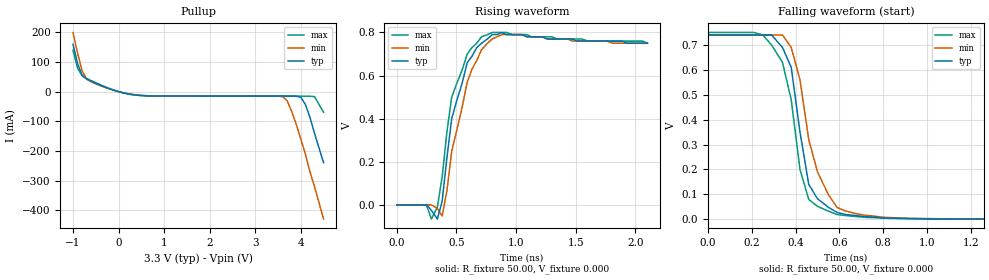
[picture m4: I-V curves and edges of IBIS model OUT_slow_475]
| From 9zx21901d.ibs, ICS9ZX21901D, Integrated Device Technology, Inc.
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|   Model OUT_slow_475
[Model]   OUT_slow_475
Model_type   Open_source
Polarity   Non-Inverting
Enable   Active-High
Vmeas =  0.350V
Cref =   2.00pF
Rref =  83.000
Vref =   0.350V
C_comp   3.40pF   2.85pF   3.95pF
[Temperature Range]   27.00   70.00   0.000
[Voltage Range]   3.30V   3.00V   3.60V
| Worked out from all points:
|   slope of the pullup table from 0 to 0.495 V, typ, clamps not added: 38 ohm
|   rising waveform, R_fixture 50.00, V_fixture 0.000: 20-80 % time 157ps typ, 172ps min, 145ps max; typ from 0.001 V to 0.75 V
|   falling waveform, R_fixture 50.00, V_fixture 0.000: 20-80 % time 75.6ps typ, 113ps min, 88.4ps max; typ from 0.74 V to 0.001 V
[Pullup]
| voltage   I(typ)   I(min)   I(max)
| -3.30   2.07A   2.09A   2.05A
| -3.10   1.90A   1.92A   1.88A
| -2.90   1.73A   1.75A   1.71A
| -2.70   1.56A   1.58A   1.54A
| -2.50   1.39A   1.42A   1.37A
| -2.30   1.22A   1.25A   1.20A
| -2.10   1.05A   1.08A   1.03A
| -1.90   0.89A   0.92A   0.87A
| -1.70   0.72A   0.75A   0.70A
| -1.50   0.56A   0.59A   0.53A
-1V       160mA      200mA      140mA
-900mV    95.74mA    130mA      79.64mA
-800mV    55.08mA    70.81mA    53.91mA
-700mV    42.76mA    42.1mA     45.09mA
-100mV    4.89mA     4.52mA     5.18mA
600mV     -13.67mA   -13.38mA   -13.83mA
3.6V      -14.91mA   -16.65mA   -14.97mA
3.8V      -14.95mA   -66.77mA   -14.97mA
4V        -18.98mA   -160mA     -14.97mA
4.1V      -42.81mA   -210mA     -14.99mA
4.3V      -140mA     -320mA     -16.63mA
4.5V      -240mA     -430mA     -69.57mA
|  4.70   -0.35A   -0.54A   -0.17A
|  4.90   -0.47A   -0.65A   -0.28A
|  5.10   -0.58A   -0.76A   -0.40A
|  5.30   -0.70A   -0.88A   -0.51A
|  5.50   -0.81A   -0.99A   -0.63A
|  5.70   -0.92A   -1.10A   -0.75A
|  5.90   -1.04A   -1.21A   -0.86A
|  6.10   -1.15A   -1.33A   -0.98A
|  6.60   -1.44A   -1.61A   -1.27A
[Ramp]
| variable   typ   min   max
dV/dt_r   0.45/0.16n   0.45/0.17n   0.45/0.16n
dV/dt_f   0.45/96.18p   0.45/0.11n   0.45/89.65p
R_load = 50.00
[Rising Waveform]
R_fixture = 50.00
V_fixture = 0.000
V_fixture_min = 0.000
V_fixture_max = 0.000
| time   V(typ)   V(min)   V(max)
0s        660uV      570uV      720uV
250ps     2.43mV     1.54mV     -1.71mV
290ps     -24.3mV    1.49mV     -64.21mV
340ps     -64.26mV   -14.82mV   -7.4mV
380ps     17.5mV     -50.47mV   130mV
460ps     400mV      250mV      500mV
590ps     660mV      570mV      700mV
710ps     750mV      720mV      780mV
880ps     800mV      790mV      800mV
2.1ns     750mV      750mV      750mV
[Falling Waveform]
R_fixture = 50.00
V_fixture = 0.000
V_fixture_min = 0.000
V_fixture_max = 0.000
| time   V(typ)   V(min)   V(max)
0s        740mV      740mV      750mV
250ps     740mV      740mV      740mV
340ps     690mV      740mV      630mV
380ps     610mV      690mV      480mV
420ps     350mV      560mV      200mV
460ps     140mV      320mV      79.27mV
550ps     47.75mV    98.35mV    32.35mV
590ps     27.08mV    46.41mV    18.89mV
800ps     5.5mV      7.95mV     4.11mV
2.1ns     660uV      580uV      720uV
